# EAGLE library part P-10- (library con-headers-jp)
HEADER PLUG PINS
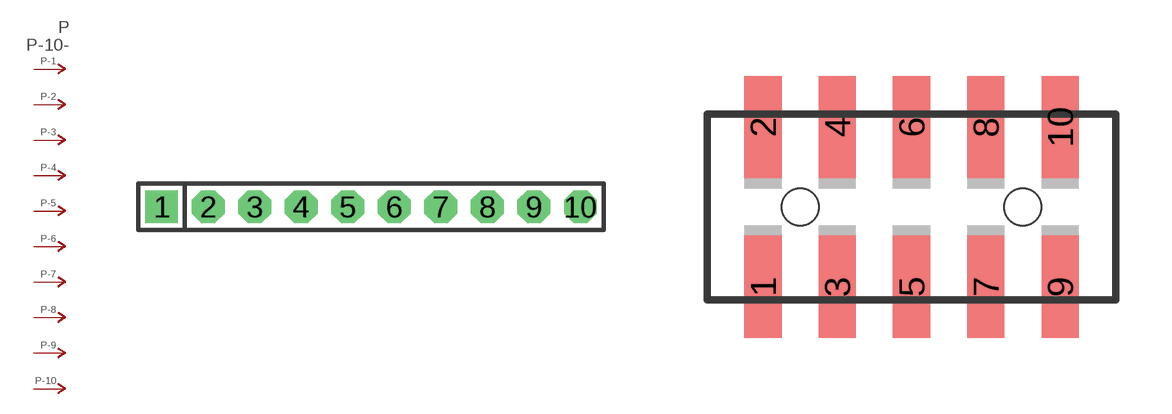
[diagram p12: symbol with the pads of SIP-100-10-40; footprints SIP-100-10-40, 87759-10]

Designator prefix P; gates -2=P-N -3=P-N -4=P-N -5=P-N -6=P-N -7=P-N -8=P-N -9=P-N -10=P-N -1=P-NV

## P-10-SIP-100-40  [SIP-100-10-40]
1  -1:P  pas
2  -2:P  pas
3  -3:P  pas
4  -4:P  pas
5  -5:P  pas
6  -6:P  pas
7  -7:P  pas
8  -8:P  pas
9  -9:P  pas
10  -10:P  pas

## P-10-87759  [87759-10]
Pads as for SIP-100-10-40

## P-10-100-2X05  [DIL-100-2X05]
Pads as for SIP-100-10-40

## P-10-100-2X05_M  [DIL-100-2X05_M]
Pads as for SIP-100-10-40

## P-10-2MM-2X05  [DIL-2MM-2X05]
Pads as for SIP-100-10-40

## P-10-2MM-2X05_M  [DIL-2MM-2X05_M]
Pads as for SIP-100-10-40

## P-10-SIP-100-32  [SIP-100-10-32]
Pads as for SIP-100-10-40

## P-10-SIP-100-40Y  [SIP-100-10-40Y]
Pads as for SIP-100-10-40

## P-10-SIP-100-32Y  [SIP-100-10-32Y]
Pads as for SIP-100-10-40

## P-10-87759_M  [87759-10_M]
Pads as for SIP-100-10-40

## P-10-LCW-110-XX-X-S  [LCW-110-XX-X-S]
Pads as for SIP-100-10-40

## P-10-LCW-110-XX-X-S-RE  [LCW-110-XX-X-S-RE]
Pads as for SIP-100-10-40

## Footprint SIP-100-10-40 (pad centres in mm)
SIP Header - 0.1", 40 mil drill
drill 1.016 pad 1.778 square: 1 -11.43,0
drill 1.016 pad 1.778 octagon: 2 -8.89,0; 3 -6.35,0; 4 -3.81,0; 5 -1.27,0; 6 1.27,0; 7 3.81,0; 8 6.35,0; 9 8.89,0; 10 11.43,0

## Footprint 87759-10 (pad centres in mm)
Molex PCB Pin Headers 2.00mm (.079") Pitch Milli-Grid Header, Vertical SMD
smd 1 x 2.75: 1 -4,-2.15; 2 -4,2.15; 3 -2,-2.15; 4 -2,2.15; 5 0,-2.15; 6 0,2.15; 7 2,-2.15; 8 2,2.15; 9 4,-2.15; 10 4,2.15
hole 1 at -3,0
hole 1 at 3,0

## Footprint DIL-100-2X05 (pad centres in mm)
PIN HEADER - 0.1"
drill 1.016 square: 1 -5.08,-1.27
drill 1.016 octagon: 2 -5.08,1.27; 3 -2.54,-1.27; 4 -2.54,1.27; 5 0,-1.27; 6 0,1.27; 7 2.54,-1.27; 8 2.54,1.27; 9 5.08,-1.27; 10 5.08,1.27

## Footprint DIL-100-2X05_M (pad centres in mm)
PIN HEADER - MIRRORED 0.1"
drill 1.016 square: 1 -5.08,1.27
drill 1.016 octagon: 2 -5.08,-1.27; 3 -2.54,1.27; 4 -2.54,-1.27; 5 0,1.27; 6 0,-1.27; 7 2.54,1.27; 8 2.54,-1.27; 9 5.08,1.27; 10 5.08,-1.27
